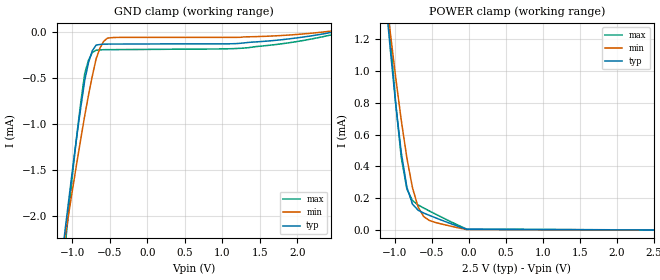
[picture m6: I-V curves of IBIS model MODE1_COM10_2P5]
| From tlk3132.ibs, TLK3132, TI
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|   Model Cell MODE1_COM10_2P5
|MODE1_COM10_2P5
[Model]   MODE1_COM10_2P5
Model_type   Input
Polarity   Non-Inverting
Vinl =  0.7V
Vinh =  1.7V
C_comp   0.5589689p   0.5151173p   0.6105178p
[Model Spec]
Vinl   0.7V   0.7V   0.7V
Vinh   1.7V   1.7V   1.7V
[Temperature Range]   25   105   0
[Voltage Range]   2.5   2.375   2.625
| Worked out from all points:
|   GND clamp passes 1 mA (typ) near -0.92 V on its own axis
|   POWER clamp passes 1 mA (typ) near -1.03 V on its own axis
[POWER_clamp]
|   voltage   I(typ)   I(min)   I(max)
-2.5V     9.469mA    7.493mA    11.61mA
-1.086V   1.284mA    1.359mA    1.393mA
-1.061V   1.154mA    1.256mA    1.232mA
-984.8mV  795.8uA    962.6uA    801.5uA
-909.1mV  488.5uA    690.9uA    456.8uA
-833.3mV  268.9uA    453.7uA    257.4uA
-757.6mV  162.6uA    266.1uA    185.1uA
-681.8mV  124.4uA    144.4uA    157.7uA
-606.1mV  106.6uA    84.37uA    138.3uA
-530.3mV  92.08uA    59.92uA    119.8uA
-25.25mV  4.064uA    2.409uA    5.396uA
2.5V      20.47nA    21.2nA     94.07nA
[GND_clamp]
|   voltage   I(typ)   I(min)   I(max)
-2.5V     -11.97mA   -9.837mA   -13.97mA
-1.136V   -2.439mA   -2.447mA   -2.677mA
-1.086V   -2.096mA   -2.182mA   -2.265mA
-1.035V   -1.758mA   -1.919mA   -1.861mA
-934.3mV  -1.109mA   -1.405mA   -1.093mA
-833.3mV  -529.3uA   -912.7uA   -453.6uA
-782.8mV  -334.1uA   -688.2uA   -309.5uA
-681.8mV  -145.4uA   -295.2uA   -201.3uA
-580.8mV  -135.3uA   -104.5uA   -195.5uA
-530.3mV  -134.7uA   -69.65uA   -195uA
1.288V    -122uA     -56.34uA   -178uA
2.449V    -7.76uA    7.1uA      -34.38uA
